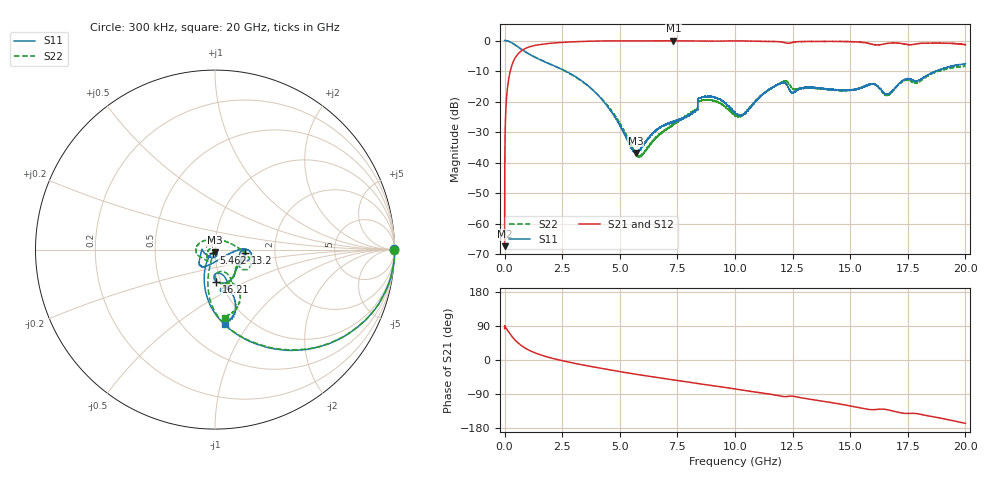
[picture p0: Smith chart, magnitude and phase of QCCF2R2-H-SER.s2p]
!QCCF2R2
!Johanson Technology Inc.
!www.johansontechnology.com
!Test Board Conditions:
!Substrate Type  RO4350B
!Substrate Thickness  10 mil
!Substrate Dk  3.66
!TL Type: GCPW
!TL Trace Width  21 mil
!TL Gap  20 mil
!Electrode orientation  Horizontal
!DUT TOPOLOGY	SERIES
!Mounting Pad LxW  16x21 mil
# MHz S  dB  R 50
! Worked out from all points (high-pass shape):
!   20001 points, 300 kHz to 20 GHz, reference 50 ohm
!   highest |S21| = -0.08 dB at 7.326 GHz (marker M1); lowest = -67.4 dB at 300 kHz (marker M2)
!   |S21| within 3 dB of the highest: 783.0737 MHz to 784.288 MHz (1.214 MHz wide, 0.155 % of centre); 784.3 MHz to end of sweep
!   lowest |S11| = -36.9 dB at 5.7 GHz (marker M3), VSWR 1.03, Z = 49.8 - j1.42 ohm
!   |S11| at or under -10 dB: 2.643 GHz to 18.72 GHz (16.08 GHz wide, 151 % of centre)
!   |S22| runs from -38.2 to 0.0 dB; largest |S21 - S12| = 0.03
!   S11 on the Smith chart (normalised r, x): 300 kHz: open; 5.462 GHz: 0.98, -0.03; 13.2 GHz: 1.40, -0.05; 16.21 GHz: 0.95, -0.35; 20 GHz: 0.77, -0.78
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0.3  -0.02 0.1  -67.37 82.9  -67.75 98.7  -0.01 -0.1
101.298  -0.07 -9.0  -17.20 80.6  -17.22 80.8  -0.07 -9.1
126.298  -0.12 -11.3  -15.34 78.4  -15.36 78.5  -0.12 -11.4
446.293  -1.39 -35.9  -5.84 53.2  -5.82 53.4  -1.41 -36.0
1399.279  -5.78 -72.7  -1.49 17.1  -1.47 16.9  -5.72 -72.0
3334.25  -13.12 -104.8  -0.32 -12.3  -0.32 -12.3  -13.27 -100.3
4498.233  -21.91 -123.9  -0.12 -25.5  -0.12 -25.4  -21.62 -108.0
5462.218  -34.45 -120.2  -0.10 -35.3  -0.12 -35.3  -33.94 -123.2
5700.215  -36.87 -95.2  -0.11 -37.6  -0.12 -37.6  -37.37 -142.5
6667.2  -29.07 -77.5  -0.12 -46.6  -0.12 -46.5  -31.11 171.0
7326.19  -26.54 -110.1  -0.08 -52.4  -0.10 -52.4  -27.36 -165.9
8286.176  -23.07 -177.1  -0.13 -61.0  -0.13 -61.0  -22.78 -125.5
8647.17  -18.49 -136.7  -0.16 -64.4  -0.17 -64.3  -19.56 -171.3
10000.15  -23.57 -86.0  -0.13 -76.5  -0.15 -76.2  -24.60 107.6
12099.12  -13.81 -10.3  -0.60 -96.3  -0.65 -96.4  -13.47 -20.1
12495.11  -17.16 -10.3  -0.65 -95.3  -0.66 -95.2  -15.71 -33.9
13202.1  -15.44 -5.9  -0.31 -103.0  -0.36 -103.1  -15.51 -25.6
13334.1  -15.45 -7.5  -0.32 -104.3  -0.35 -104.3  -15.49 -26.2
16207.06  -15.00 -88.4  -1.46 -130.1  -1.42 -130.6  -15.10 -86.3
16667.05  -17.54 -80.1  -0.89 -131.9  -0.87 -132.3  -17.81 -72.1
17343.04  -12.82 -74.9  -1.14 -140.6  -1.19 -140.5  -13.16 -67.1
20000  -7.58 -82.6  -1.38 -167.1  -1.17 -165.9  -8.34 -81.4
